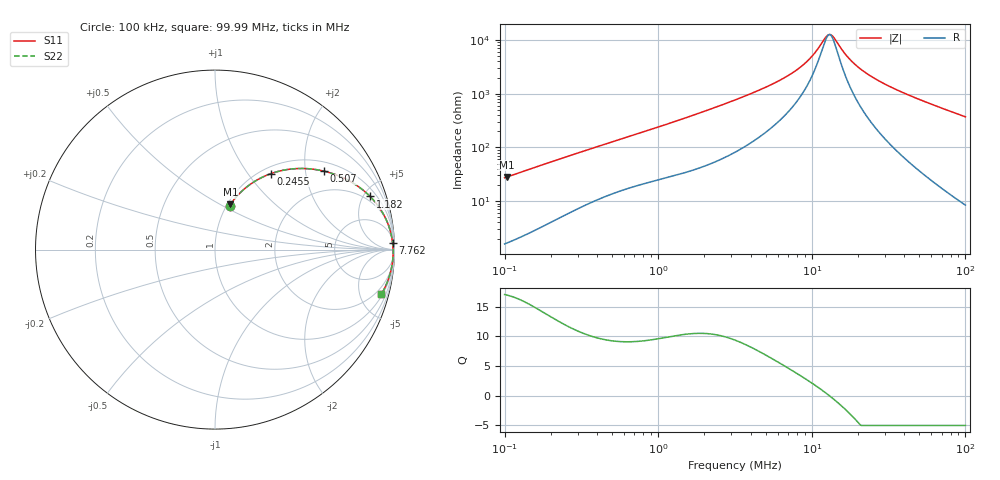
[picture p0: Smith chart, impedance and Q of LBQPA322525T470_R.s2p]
! LBQPA322525T470_R  S-PARAMETER MODEL  ( General Type )
! Model Generated by TAIYO YUDEN Corporation (http://www.ty-top.com)
! Version 1.0
! TAIYO YUDEN Control No. 191025NI43SB-FBB
! Copyright(c) 2019 TAIYO YUDEN CO.,LTD. All Rights Reserved.
! Product Description (link to TY-COMPAS)
! https://ds.yuden.co.jp/TYCOMPAS/or/detail?pn=LBQPA322525T470KR&u=M
! Products Name : Inductors
! Characteristics :
!  Inductance : 47 uH , SRF(min) : 10 MHz , DC Resistance(max) : 0.871 Ohm
!  Rated Current : Saturation :390 mA , Temp Rise : 320 mA (20 degC)
!  Case Size : 3.2 x 2.5 / 0.126 x 0.098 [mm/inch] , Thickness : 2.5 / 0.098 [mm/inch]
!  (Conditions: Temperature = 25 degC , DC Bias Current/Voltage = 0A / 0V)
! External Node Assignments :
!  1  o---GGG---o  2
! GND o---------o GND
! Frequency Range : 0.1MHz  -  99.992428MHz  [ 402 STEP ]
# MHz S RI R 50
! Freq[MHz].  S11 Real  S11 Imag  S21 Real  S21 Imag  S12 Real  S12 Imag  S22 Real  S22 Imag
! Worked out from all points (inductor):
!   401 points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, 100 kHz to 99.99 MHz, reference 50 ohm
!   read as one part in series: L = 43.1 uH near 103.5 kHz
!   highest Q = 16.9 at 103.5 kHz (marker M1), where L = 43.2 uH
!   self-resonance near 12.81 MHz
!   S11 on the Smith chart (normalised r, x): 100 kHz: 1.03, +0.54; 245.5 kHz: 1.11, +1.30; 507 kHz: 1.28, +2.54; 1.182 MHz: 1.56, +5.57; 7.762 MHz: 14, +51; 99.99 MHz: 1.17, -7.41
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0.1  0.0814 0.2456  0.9186 -0.2456  0.9186 -0.2456  0.0814 0.2456
0.103514  0.0862 0.2526  0.9138 -0.2526  0.9138 -0.2526  0.0862 0.2526
0.159403  0.1722 0.3452  0.8278 -0.3452  0.8278 -0.3452  0.1722 0.3452
0.245468  0.3126 0.4236  0.6874 -0.4236  0.6874 -0.4236  0.3126 0.4236
0.318049  0.4169 0.4481  0.5831 -0.4481  0.5831 -0.4481  0.4169 0.4481
0.506982  0.6089 0.4367  0.3911 -0.4367  0.3911 -0.4367  0.6089 0.4367
1.011554  0.8296 0.3275  0.1704 -0.3275  0.1704 -0.3275  0.8296 0.3275
1.181648  0.8638 0.2962  0.1362 -0.2962  0.1362 -0.2962  0.8638 0.2962
1.85134  0.932 0.2085  0.068 -0.2085  0.068 -0.2085  0.932 0.2085
3.162158  0.9703 0.1246  0.0297 -0.1246  0.0297 -0.1246  0.9703 0.1246
5.401085  0.9851 0.066  0.0149 -0.066  0.0149 -0.066  0.9851 0.066
7.762101  0.9894 0.0363  0.0106 -0.0363  0.0106 -0.0363  0.9894 0.0363
10.05722  0.9912 0.0177  0.00883 -0.0177  0.00883 -0.0177  0.9912 0.0177
12.37306  0.992 0.00347  0.00798 -0.00347  0.00798 -0.00347  0.992 0.00347
13.25796  0.9922 -0.00125  0.00779 0.00125  0.00779 0.00125  0.9922 -0.00125
13.96293  0.9923 -0.00481  0.00769 0.00481  0.00769 0.00481  0.9923 -0.00481
16.88401  0.9924 -0.0181  0.00757 0.0181  0.00757 0.0181  0.9924 -0.0181
19.38541  0.9922 -0.0283  0.00776 0.0283  0.00776 0.0283  0.9922 -0.0283
24.26464  0.9913 -0.0461  0.00872 0.0461  0.00872 0.0461  0.9913 -0.0461
31.98693  0.9886 -0.0714  0.0114 0.0714  0.0114 0.0714  0.9886 -0.0714
53.69948  0.9756 -0.1341  0.0244 0.1341  0.0244 0.1341  0.9756 -0.1341
99.99243  0.9273 -0.2485  0.0727 0.2485  0.0727 0.2485  0.9273 -0.2485
